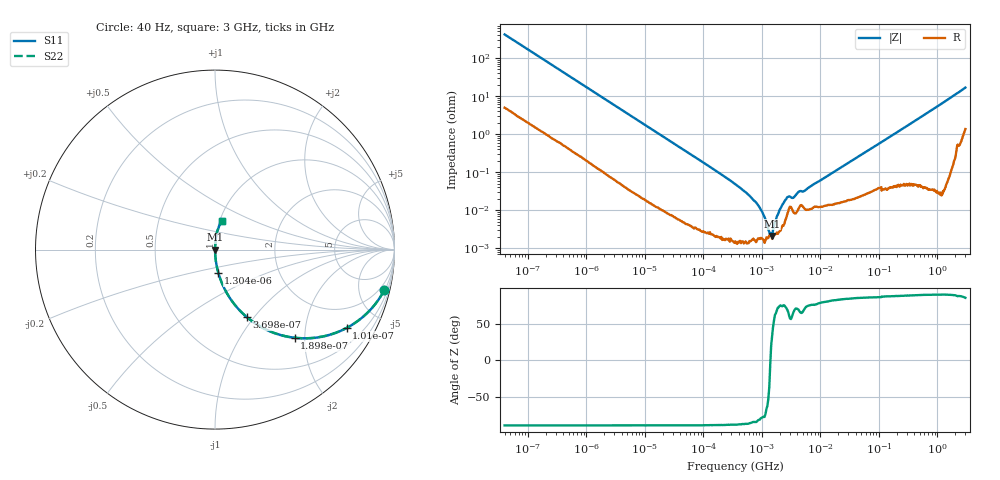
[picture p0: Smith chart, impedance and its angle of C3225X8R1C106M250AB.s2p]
! S-parameter Generated by TDK Corporation
! Copyright(C) 2015 TDK Corporation.
! All Rights Reserved.
! TDK P/N: C3225X8R1C106M250AB (Multilayer Ceramic Chip Capacitors)
! Property: C=10uF
! Size(LxWxT): 3.2x2.5x2.5mm, 0.126x0.098x0.098inches
! Model Type: s2p (Touchstone File Format Version 1.0)
! Frequency: DC=Yes Start=0.00004MHz Stop=3000MHz 568points Log-sweep
! Note: This model was converted from impedance.
! Model Generated on Jun. 23, 2015
! Hash(MD5):
! Port Assignments:
!  1 ---| |--- 2
! Applicable Conditions:
!  Temperature = 25 degC
!  DC Bias Voltage = 0 V
!  Small Signal Operation
! Terms and conditions regarding TDK Simulation Models
! (1)This simulation model is being provided solely for informational purposes. Please refer to the specifications of the products in terms of detailed characteristics of such products.
! (2)In no event shall TDK Corporation of any of its subsidiaries be liable for any loss or damage arising, directly or indirectly,
!  From any information contained in this simulation model, including, but not limited to loss or damages arising from any inaccuracies, omissions or errors in connection with such information.
! (3)Any and all copyrights on this simulation model are owned by TDK Corporation.
!  Duplication or redistribution of this simulation model without prior written permission from TDK Corporation is prohibited.
! (4)This simulation model is subject to any modification or change without any prior notice.
! (5)Neither TDK Corporation nor any of its subsidiaries shall make any warranty, express or implied,
!  Including but not limited to the correctness, implied warranties of merchantability and fitness for a particular purpose with respect to this simulation models.
! (6)The use of this simulation model shall be deemed to have consented to the terms and conditions hereof.
# MHz S MA R 50
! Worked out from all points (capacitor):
!   567 points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, 40 Hz to 3 GHz, reference 50 ohm
!   read as one part in series: C = 9.51 uF near 43.08 Hz
!   lowest |Z| = 2.1 mohm at 1.493 MHz (marker M1)
!   series resonance near 1.397 MHz, so ESL is about 1.4 nH
!   S11 on the Smith chart (normalised r, x): 40 Hz: 1.10, -8.32; 101 Hz: 1.04, -3.34; 189.8 Hz: 1.02, -1.79; 369.8 Hz: 1.01, -0.92; 1.304 kHz: 1.00, -0.26; 3 GHz: 1.03, +0.33
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4e-05  0.9697 -13.5  0.233 75.8  0.233 75.8  0.9697 -13.5
6.4765e-05  0.9293 -21.0  0.3586 68.3  0.3586 68.3  0.9293 -21.0
0.000101046  0.8532 -30.8  0.5115 58.6  0.5115 58.6  0.8532 -30.8
0.000189754  0.662 -47.9  0.7416 41.4  0.7416 41.4  0.662 -47.9
0.000369794  0.4165 -64.7  0.9041 24.6  0.9041 24.6  0.4165 -64.7
0.00083584  0.2009 -77.7  0.9772 11.6  0.9772 11.6  0.2009 -77.7
0.001304077  0.1311 -81.8  0.9899 7.5  0.9899 7.5  0.1311 -81.8
0.003681768  0.04733 -86.7  0.9984 2.7  0.9984 2.7  0.04733 -86.7
0.01746572  0.0101 -88.8  0.9998 0.6  0.9998 0.6  0.0101 -88.8
0.3516829  0.0004798 -88.2  1 0.0  1 0.0  0.0004798 -88.2
0.5909189  0.0002529 -86.9  1 0.0  1 0.0  0.0002529 -86.9
0.9928978  9.451e-05 -78.8  1 0.0  1 0.0  9.451e-05 -78.8
1.492747  2.096e-05 33.4  1 -0.0  1 -0.0  2.096e-05 33.4
1.934971  8.672e-05 72.3  1 -0.0  1 -0.0  8.672e-05 72.3
2.701217  0.0002173 69.3  0.9999 -0.0  0.9999 -0.0  0.0002173 69.3
3.501449  0.0002157 66.6  0.9999 -0.0  0.9999 -0.0  0.0002157 66.6
4.214436  0.0003025 69.1  0.9999 -0.0  0.9999 -0.0  0.0003025 69.1
5.264165  0.0003172 69.1  0.9999 -0.0  0.9999 -0.0  0.0003172 69.1
7.348767  0.0004613 75.7  0.9999 -0.0  0.9999 -0.0  0.0004613 75.7
149.005  0.008239 86.9  0.9996 -0.5  0.9996 -0.5  0.008239 86.9
939.5906  0.05033 86.8  0.9984 -2.9  0.9984 -2.9  0.05033 86.8
3000  0.1628 76.0  0.9735 -9.3  0.9735 -9.3  0.1628 76.0
